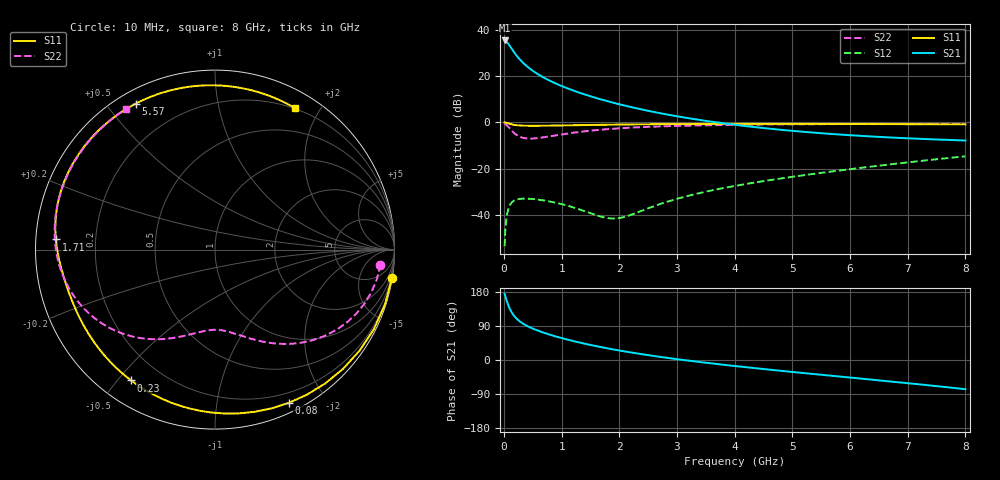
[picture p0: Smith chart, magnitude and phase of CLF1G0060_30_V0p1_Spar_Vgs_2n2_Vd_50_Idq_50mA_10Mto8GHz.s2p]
! Created Wed Apr  4 15:50:08 2012
# ghz S ma R 50
! 2 Port Network Data from SP1.SP block
! freq  magS11  angS11  magS21  angS21  magS12  angS12  magS22  angS22
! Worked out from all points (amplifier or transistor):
!   800 points, 10 MHz to 8 GHz, reference 50 ohm
!   highest |S21| = 35.3 dB at 10 MHz (marker M1)
!   |S21| within 3 dB of that: start of sweep to 116.7 MHz
!   unconditionally stable (mu >= 1): 1.478 GHz to 2.471 GHz
!   at 1.34 GHz: K = 0.82, MSG = 25.2 dB, |S12| = -37.8 dB
!   at 4.01 GHz: K = 0.33, MSG = 13.2 dB, |S12| = -27.4 dB
!   at 8 GHz: K = 0.34, MSG = 3.4 dB, |S12| = -14.7 dB
!   S11 on the Smith chart (normalised r, x): 10 MHz: 0, -13; 80 MHz: 0.09, -1.58; 230 MHz: 0.09, -0.54; 1.71 GHz: 0.06, +0.03; 5.57 GHz: 0.05, +0.59; 8 GHz: 0.19, +1.70
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0.01  0.9987 -9.0  58.52 174.6  0.002134 84.9  0.9257 -5.2
0.04  0.983 -34.9  55.55 159.4  0.008099 70.1  0.8849 -20.0
0.06  0.966 -50.5  52.2 150.3  0.01141 61.3  0.8395 -28.9
0.08  0.9477 -64.4  48.38 142.2  0.01409 53.5  0.7885 -36.7
0.09  0.9387 -70.6  46.44 138.6  0.01521 50.1  0.7627 -40.2
0.11  0.9222 -81.8  42.64 132.1  0.01706 43.9  0.7134 -46.4
0.15  0.8958 -99.6  35.93 121.6  0.01955 34.1  0.6294 -56.4
0.19  0.8778 -112.7  30.56 113.7  0.021 26.8  0.567 -63.9
0.23  0.8659 -122.6  26.36 107.4  0.02184 21.2  0.5227 -69.8
0.29  0.8549 -133.5  21.66 99.9  0.02246 14.8  0.4807 -76.8
0.37  0.8478 -143.4  17.34 92.3  0.02265 8.6  0.4539 -83.9
0.48  0.8447 -152.3  13.46 84.1  0.02231 2.4  0.4474 -91.6
0.61  0.8457 -159.2  10.53 76.2  0.02142 -3.0  0.4621 -99.0
0.92  0.8557 -169.3  6.694 61.1  0.01819 -10.6  0.5305 -113.1
1.35  0.8742 -177.9  4.192 44.6  0.01273 -10.2  0.6312 -128.2
1.71  0.8884 176.3  3.059 33.1  0.00906 7.3  0.7002 -138.4
2.68  0.9142 162.6  1.601 8.8  0.01686 68.2  0.817 -159.3
4.01  0.9273 144.1  0.8846 -16.0  0.04274 64.1  0.8865 179.9
5.34  0.9265 122.7  0.6041 -36.6  0.07664 47.7  0.9143 162.2
5.57  0.9254 118.5  0.5745 -40.0  0.08364 44.4  0.917 159.2
6.67  0.9175 95.8  0.474 -56.2  0.1232 26.4  0.9248 144.0
8  0.9057 60.5  0.406 -77.0  0.1851 -1.1  0.9267 122.5
